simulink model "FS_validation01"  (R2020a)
settings: Solver=ode45  StartTime=0.0  StopTime=2000  RelTol=1e-3  EnableMultiTasking=on
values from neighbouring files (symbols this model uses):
  Ts = 0.2    [init_model.m]
libraries: fuzblock x1

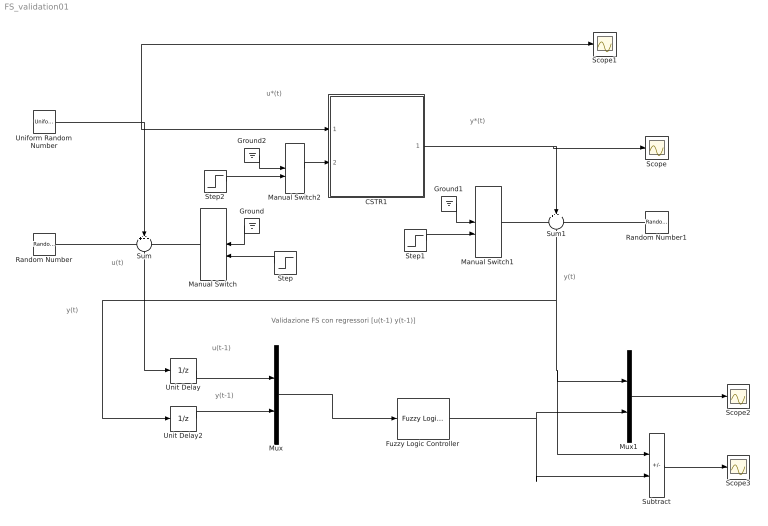
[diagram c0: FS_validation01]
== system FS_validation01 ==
  note: u(t)
  note: u*(t)
  note: y(t)
  note: y*(t)
  note: Validazione FS con regressori [u(t-1) y(t-1)]
  note: u(t-1)
  note: y(t)
  note: y(t-1)
  CSTR1 : Subsystem
  Fuzzy Logic Controller : fuzblock/Fuzzy Logic  Controller  FIS=FIS01  OutputSampleNumber=101  DataType=double  FuzzifiedInputs=off  RuleFiringStrengths=off  RuleOutputs=off  AggregatedOutputs=off  SimulateUsing=Interpreted execution  OutOfRangeInputValueMessage=warning  NoRuleFiredMessage=warning  EmptyOutputFuzzySetMessage=warning
  Ground : Ground
  Ground1 : Ground
  Ground2 : Ground
  Manual Switch : ManualSwitch
  Manual Switch1 : ManualSwitch
  Manual Switch2 : ManualSwitch
  Mux : Mux  Inputs=2
  Mux1 : Mux  Inputs=2
  Random Number : RandomNumber  Variance=0.0001  Seed=1  SampleTime=Ts
  Random Number1 : RandomNumber  Variance=0.0005  Seed=2  SampleTime=Ts
  Scope{,1..3} (4 alike) : Scope
  Step : Step  Time=1000  After=10  SampleTime=0
  Step1 : Step  Time=1000  After=10  SampleTime=0
  Step2 : Step  Time=1000  SampleTime=0
  Subtract : Sum  Inputs=+-
  Sum : Sum  Inputs=+++  SaturateOnIntegerOverflow=on
  Sum1 : Sum  Inputs=+++  SaturateOnIntegerOverflow=on
  Uniform Random Number : UniformRandomNumber  Minimum=0  Maximum=4  SampleTime=20
  Unit Delay : UnitDelay  SampleTime=Ts  HasFrameUpgradeWarning=on
  Unit Delay2 : UnitDelay  SampleTime=Ts  HasFrameUpgradeWarning=on
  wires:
  Uniform Random Number/1 -> CSTR1/1(w), Scope1/1, Sum/2
  Random Number/1 -> Sum/1
  Manual Switch/1 -> Sum/3
  Sum/1 -> Unit Delay/1
  Ground/1 -> Manual Switch/1
  Step/1 -> Manual Switch/2
  Ground1/1 -> Manual Switch1/1
  Step1/1 -> Manual Switch1/2
  CSTR1/1(Cb) -> Scope/1, Sum1/2
  Manual Switch1/1 -> Sum1/1
  Random Number1/1 -> Sum1/3
  Sum1/1 -> Subtract/1, Mux1/1, Unit Delay2/1
  Step2/1 -> Manual Switch2/2
  Manual Switch2/1 -> CSTR1/2(f)
  Ground2/1 -> Manual Switch2/1
  Unit Delay2/1 -> Mux/2
  Unit Delay/1 -> Mux/1
  Mux/1 -> Fuzzy Logic Controller/1
  Fuzzy Logic Controller/1 -> Subtract/2, Mux1/2
  Mux1/1 -> Scope2/1
  Subtract/1 -> Scope3/1

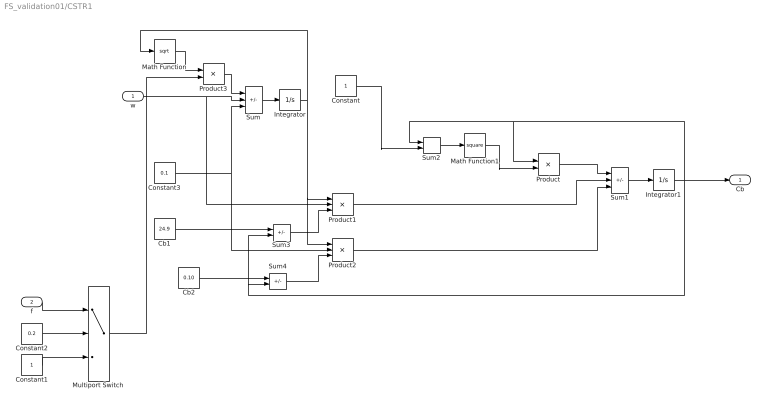
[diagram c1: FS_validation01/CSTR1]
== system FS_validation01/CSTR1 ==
  w : Inport
  f : Inport  Port=2
  Cb1 : Constant  Value=24.9
  Cb2 : Constant  Value=0.10
  Constant : Constant
  Constant1 : Constant
  Constant2 : Constant  Value=0.2
  Constant3 : Constant  Value=0.1
  Integrator : Integrator  InitialCondition=30  LimitOutput=on  LowerSaturationLimit=1
  Integrator1 : Integrator  InitialCondition=22
  Math Function : Math  Operator=sqrt
  Math Function1 : Math  Operator=square
  Multiport Switch : MultiPortSwitch  DataPortOrder=Zero-based contiguous  Inputs=2  zeroidx=on
  Product : Product  Inputs=*/  SaturateOnIntegerOverflow=on
  Product1 : Product  Inputs=/**  SaturateOnIntegerOverflow=on
  Product2 : Product  Inputs=/**  SaturateOnIntegerOverflow=on
  Product3 : Product
  Sum : Sum  Inputs=-++  SaturateOnIntegerOverflow=on
  Sum1 : Sum  Inputs=-++  SaturateOnIntegerOverflow=on
  Sum2 : Sum  SaturateOnIntegerOverflow=on
  Sum3 : Sum  Inputs=+-  SaturateOnIntegerOverflow=on
  Sum4 : Sum  Inputs=+-  SaturateOnIntegerOverflow=on
  Cb : Outport
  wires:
  Sum/1 -> Integrator/1
  Product3/1 -> Sum/1
  Math Function/1 -> Product3/1
  Integrator/1 -> Math Function/1, Product1/1, Product2/1
  Sum3/1 -> Product1/3
  Sum4/1 -> Product2/3
  Sum2/1 -> Math Function1/1
  Sum1/1 -> Integrator1/1
  Math Function1/1 -> Product/2
  Product/1 -> Sum1/1
  Product1/1 -> Sum1/2
  Product2/1 -> Sum1/3
  w/1 -> Sum/2, Product1/2
  Constant3/1 -> Product2/2, Sum/3
  Integrator1/1 -> Sum3/2, Sum4/2, Sum2/1, Product/1, Cb/1
  Constant1/1 -> Multiport Switch/3
  f/1 -> Multiport Switch/1
  Constant2/1 -> Multiport Switch/2
  Cb2/1 -> Sum4/1
  Cb1/1 -> Sum3/1
  Constant/1 -> Sum2/2
  Multiport Switch/1 -> Product3/2
